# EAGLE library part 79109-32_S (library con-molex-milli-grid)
RECEPTACAL
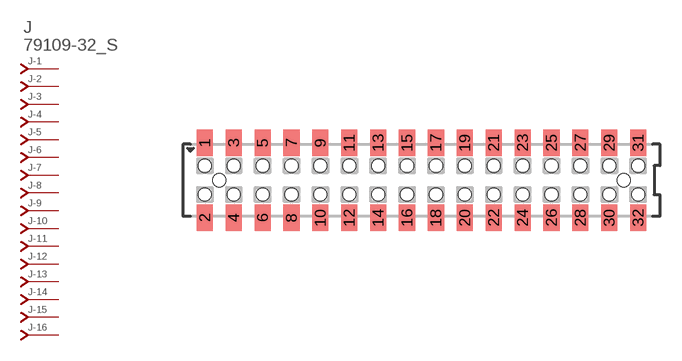
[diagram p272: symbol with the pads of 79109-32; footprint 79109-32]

Designator prefix J; gates -1=J-NV -2=J-N -3=J-N -4=J-N -5=J-N -6=J-N -7=J-N -8=J-N -9=J-N -10=J-N -11=J-N -12=J-N -13=J-N -14=J-N -15=J-N -16=J-N -17=J-N -18=J-N -19=J-N -20=J-N -21=J-N -22=J-N -23=J-N -24=J-N -25=J-N -26=J-N -27=J-N -28=J-N -29=J-N -30=J-N -31=J-N -32=J-N

## 79109-32_S  [79109-32]
1  -1:J  pas
2  -2:J  pas
3  -3:J  pas
4  -4:J  pas
5  -5:J  pas
6  -6:J  pas
7  -7:J  pas
8  -8:J  pas
9  -9:J  pas
10  -10:J  pas
11  -11:J  pas
12  -12:J  pas
13  -13:J  pas
14  -14:J  pas
15  -15:J  pas
16  -16:J  pas
17  -17:J  pas
18  -18:J  pas
19  -19:J  pas
20  -20:J  pas
21  -21:J  pas
22  -22:J  pas
23  -23:J  pas
24  -24:J  pas
25  -25:J  pas
26  -26:J  pas
27  -27:J  pas
28  -28:J  pas
29  -29:J  pas
30  -30:J  pas
31  -31:J  pas
32  -32:J  pas

## Footprint 79109-32 (pad centres in mm)
RECEPTACAL SMD Dual Row, Vertical, Pass-Thru
smd 1.12 x 1.83: 1 -15,2.6; 2 -15,-2.6; 3 -13,2.6; 4 -13,-2.6; 5 -11,2.6; 6 -11,-2.6; 7 -9,2.6; 8 -9,-2.6; 9 -7,2.6; 10 -7,-2.6; 11 -5,2.6; 12 -5,-2.6; 13 -3,2.6; 14 -3,-2.6; 15 -1,2.6; 16 -1,-2.6; 17 1,2.6; 18 1,-2.6; 19 3,2.6; 20 3,-2.6; 21 5,2.6; 22 5,-2.6; 23 7,2.6; 24 7,-2.6; 25 9,2.6; 26 9,-2.6; 27 11,2.6; 28 11,-2.6; 29 13,2.6; 30 13,-2.6; 31 15,2.6; 32 15,-2.6
hole 0.914 at -14,0
hole 0.914 at -15,1
hole 0.914 at -15,-1
hole 0.914 at -13,-1
hole 0.914 at -13,1
hole 0.914 at -11,-1
hole 0.914 at -11,1
hole 0.914 at 14,0
hole 0.914 at -9,1
hole 0.914 at -9,-1
hole 0.914 at -7,1
hole 0.914 at -7,-1
hole 0.914 at -5,1
hole 0.914 at -5,-1
hole 0.914 at -3,1
hole 0.914 at -3,-1
hole 0.914 at -1,-1
hole 0.914 at -1,1
hole 0.914 at 1,1
hole 0.914 at 1,-1
hole 0.914 at 3,1
hole 0.914 at 3,-1
hole 0.914 at 5,1
hole 0.914 at 5,-1
hole 0.914 at 7,-1
hole 0.914 at 7,1
hole 0.914 at 9,1
hole 0.914 at 11,1
hole 0.914 at 13,1
hole 0.914 at 9,-1
hole 0.914 at 11,-1
hole 0.914 at 13,-1
hole 0.914 at 15,-1
hole 0.914 at 15,1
